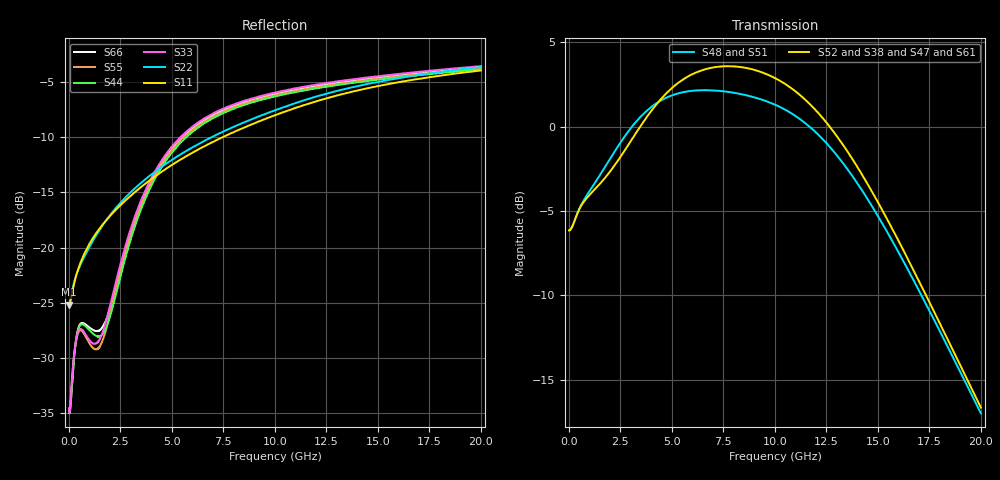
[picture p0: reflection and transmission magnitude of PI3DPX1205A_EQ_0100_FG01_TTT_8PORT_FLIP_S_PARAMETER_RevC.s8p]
! NPort=8 DATA=2000 NOISE=0 GROUPDELAY=0 COMPLEX_DATAFORMAT=POLAR
! NumOfBlock=1 NumOfParam=0
! .MODEL Smodel S TSTONEFILE=PI3DPX1205A_EQ_0100_FG01_TTT_8PORT_FLIP_S_PARAMETER_RevC.s8p TYPE=S
!  -- The above .MODEL line can be used for the S element in the netlist.
! The s parameter is extracted from the linear redriver, it is not bi-directional;
! only s(5,1)s(6,2)s(3,7)s(4,8) should be the insertion loss
!  Port definition:
!  Port1 = AIP
!  Port2 = AIN
!  Port3 = BOP
!  Port4 = BON
!  Port5 = AOP
!  Port6 = AON
!  Port7 = BIP
!  Port8 = BIN
# Hz S MA R  50
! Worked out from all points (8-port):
!   2000 points, 10 MHz to 20 GHz, reference 50 ohm
!   strongest paths, dB at 10 MHz, 5.01 GHz, 10.01 GHz, 15.01 GHz, 20 GHz:
!     S52: -6.1, 2.3, 2.9, -4.5, -16.7
!     S38: -6.1, 2.3, 2.9, -4.5, -16.7
!     S47: -6.1, 2.3, 2.9, -4.5, -16.6
!     S61: -6.1, 2.3, 2.9, -4.5, -16.6
!     S48: -6.1, 1.9, 1.3, -5.3, -17.0
!     S51: -6.1, 1.8, 1.3, -5.3, -17.0
!   lowest |S11| = -25.2 dB at 10 MHz (marker M1), VSWR 1.12, Z = 44.8 - j0.115 ohm
!   |S11| at or under -10 dB: start of sweep to 7.467 GHz
